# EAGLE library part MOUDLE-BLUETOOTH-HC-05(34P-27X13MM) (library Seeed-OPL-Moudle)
317030002
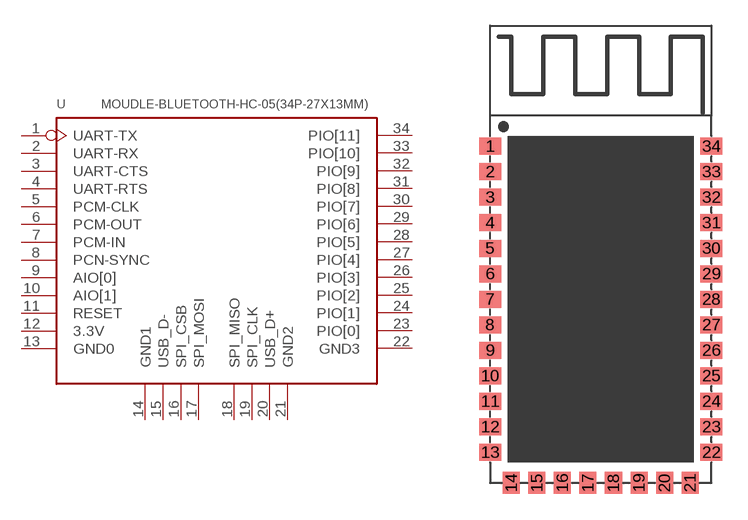
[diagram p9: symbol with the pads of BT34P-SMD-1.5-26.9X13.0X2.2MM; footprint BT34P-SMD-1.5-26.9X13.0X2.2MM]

Designator prefix U

## MOUDLE-BLUETOOTH-HC-05(34P-27X13MM) (MPN: HC-05; VALUE: HC-05(34P 27X13MM))  [BT34P-SMD-1.5-26.9X13.0X2.2MM]
1  UART-TX
2  UART-RX
3  UART-CTS
4  UART-RTS
5  PCM-CLK
6  PCM-OUT
7  PCM-IN
8  PCN-SYNC
9  AIO[0]
10  AIO[1]
11  RESET
12  3.3V
13  GND0
14  GND1
15  USB_D-
16  SPI_CSB
17  SPI_MOSI
18  SPI_MISO
19  SPI_CLK
20  USB_D+
21  GND2
22  GND3
23  PIO[0]
24  PIO[1]
25  PIO[2]
26  PIO[3]
27  PIO[4]
28  PIO[5]
29  PIO[6]
30  PIO[7]
31  PIO[8]
32  PIO[9]
33  PIO[10]
34  PIO[11]

## Footprint BT34P-SMD-1.5-26.9X13.0X2.2MM (pad centres in mm)
smd 1.3 x 1: 1 -6.5,19.8; 2 -6.5,18.3; 3 -6.5,16.8; 4 -6.5,15.3; 5 -6.5,13.8; 6 -6.5,12.3; 7 -6.5,10.8; 8 -6.5,9.3; 9 -6.5,7.8; 10 -6.5,6.3; 11 -6.5,4.8; 12 -6.5,3.3; 13 -6.5,1.8; 22 6.5,1.8; 23 6.5,3.3; 24 6.5,4.8; 25 6.5,6.3; 26 6.5,7.8; 27 6.5,9.3; 28 6.5,10.8; 29 6.5,12.3; 30 6.5,13.8; 31 6.5,15.3; 32 6.5,16.8; 33 6.5,18.3; 34 6.5,19.8
smd 1 x 1.3: 14 -5.25,0; 15 -3.75,0; 16 -2.25,0; 17 -0.75,0; 18 0.75,0; 19 2.25,0; 20 3.75,0; 21 5.25,0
